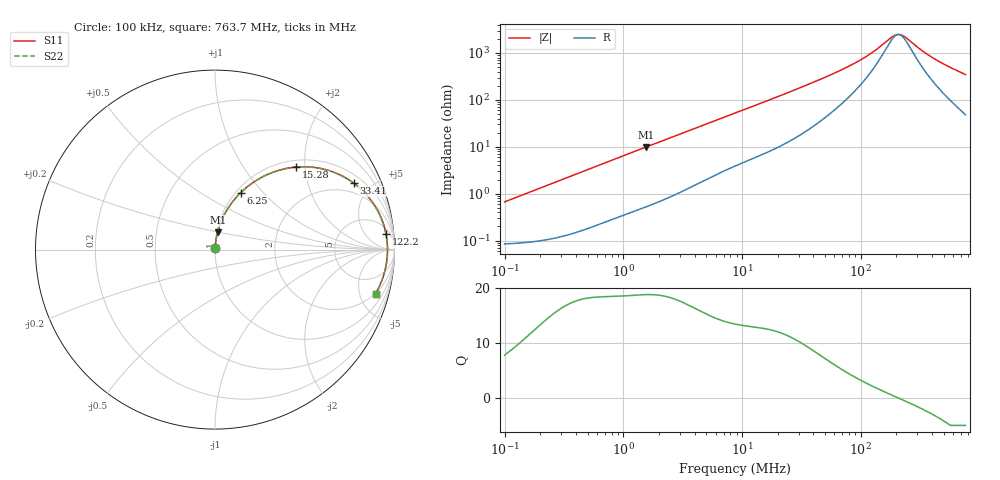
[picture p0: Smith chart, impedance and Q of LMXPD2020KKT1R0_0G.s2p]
! LMXPD2020KKT1R0_0G  S-PARAMETER MODEL  ( General Type )
! Model Generated by TAIYO YUDEN Corporation (https://www.yuden.co.jp/en/)
! Version 1.0
! TAIYO YUDEN Control No. 191023NI43SB-FBB
! Copyright(c) 2019 TAIYO YUDEN CO.,LTD. All Rights Reserved.
! Product Description (link to TY-COMPAS)
! https://ds.yuden.co.jp/TYCOMPAS/or/detail?pn=LMXPD2020KKT1R0N0G&u=M
! Products Name : Inductors
! Characteristics :
!  Inductance : 1.0 uH , SRF(min) : -Hz , DC Resistance(max) : 0.096 Ohm
!  Rated Current : Saturation :1550 mA , Temp Rise : 1600 mA (40 degC)
!  Case Size : 2.0 x 2.0 / 0.079 x 0.079 [mm/inch] , Thickness : 1 / 0.039 [mm/inch]
!  (Conditions: Temperature = 25 degC , DC Bias Current/Voltage = 0A / 0V)
! External Node Assignments :
!  1  o---GGG---o  2
! GND o---------o GND
! Frequency Range : 0.1MHz  -  763.723512MHz  [ 402 STEP ]
# MHz S RI R 50
! Freq[MHz].  S11 Real  S11 Imag  S21 Real  S21 Imag  S12 Real  S12 Imag  S22 Real  S22 Imag
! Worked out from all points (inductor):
!   401 points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, 100 kHz to 763.7 MHz, reference 50 ohm
!   read as one part in series: L = 1.06 uH near 104.6 kHz
!   highest Q = 18.8 at 1.563 MHz (marker M1), where L = 1.01 uH
!   self-resonance near 208.1 MHz
!   S11 on the Smith chart (normalised r, x): 100 kHz: 1.00, +0.01; 6.25 MHz: 1.05, +0.76; 15.28 MHz: 1.14, +1.79; 33.41 MHz: 1.40, +3.91; 122.2 MHz: 9, +18; 763.7 MHz: 1.97, -6.89
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0.1  0.000893 0.00663  0.9991 -0.00663  0.9991 -0.00663  0.000893 0.00663
0.447087  0.00249 0.0292  0.9975 -0.0292  0.9975 -0.0292  0.00249 0.0292
1.563158  0.0148 0.0972  0.9852 -0.0972  0.9852 -0.0972  0.0148 0.0972
1.998866  0.022 0.1224  0.978 -0.1224  0.978 -0.1224  0.022 0.1224
3.737568  0.0626 0.214  0.9374 -0.214  0.9374 -0.214  0.0626 0.214
6.249683  0.1428 0.3168  0.8572 -0.3168  0.8572 -0.3168  0.1428 0.3168
8.739128  0.2316 0.3863  0.7684 -0.3863  0.7684 -0.3863  0.2316 0.3863
15.28099  0.45 0.4596  0.55 -0.4596  0.55 -0.4596  0.45 0.4596
21.85089  0.6109 0.4469  0.3891 -0.4469  0.3891 -0.4469  0.6109 0.4469
33.41246  0.772 0.3712  0.228 -0.3712  0.228 -0.3712  0.772 0.3712
39.07148  0.8167 0.334  0.1833 -0.334  0.1833 -0.334  0.8167 0.334
74.70897  0.9241 0.1801  0.0759 -0.1801  0.0759 -0.1801  0.9241 0.1801
97.69241  0.9433 0.126  0.0567 -0.126  0.0567 -0.126  0.9433 0.126
122.1615  0.953 0.0857  0.047 -0.0857  0.047 -0.0857  0.953 0.0857
174.6834  0.9604 0.0272  0.0396 -0.0272  0.0396 -0.0272  0.9604 0.0272
199.7541  0.9612 0.00636  0.0388 -0.00636  0.0388 -0.00636  0.9612 0.00636
223.3739  0.9612 -0.011  0.0388 0.011  0.0388 0.011  0.9612 -0.011
244.2653  0.9607 -0.0249  0.0393 0.0249  0.0393 0.0249  0.9607 -0.0249
334.0139  0.9555 -0.0756  0.0445 0.0756  0.0445 0.0756  0.9555 -0.0756
408.4422  0.9485 -0.1111  0.0515 0.1111  0.0515 0.1111  0.9485 -0.1111
558.5131  0.9292 -0.1731  0.0708 0.1731  0.0708 0.1731  0.9292 -0.1731
763.7235  0.8944 -0.2449  0.1056 0.2449  0.1056 0.2449  0.8944 -0.2449
